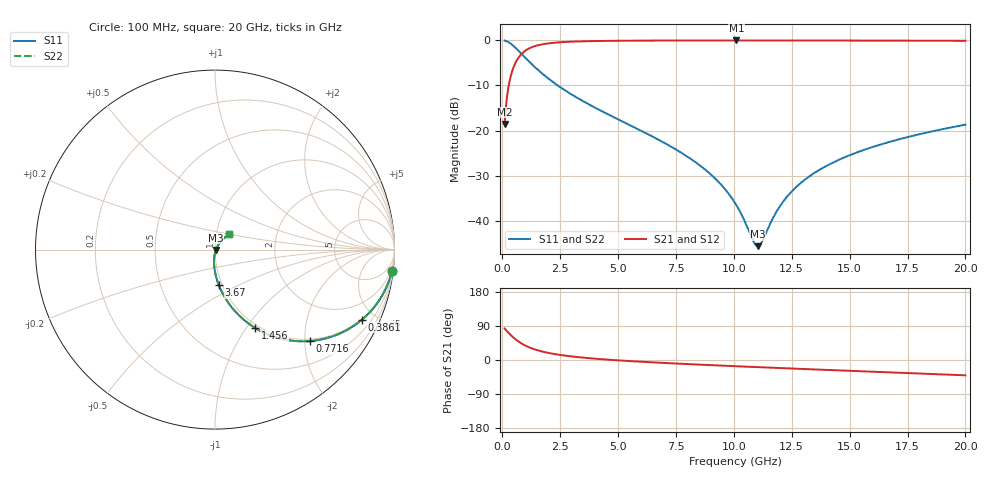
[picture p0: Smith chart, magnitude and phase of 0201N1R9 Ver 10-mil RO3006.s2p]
# GHz S MA R 50
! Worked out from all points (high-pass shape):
!   1601 points, 100 MHz to 20 GHz, reference 50 ohm
!   highest |S21| = -0.05 dB at 10.11 GHz (marker M1); lowest = -18.5 dB at 100 MHz (marker M2)
!   |S21| within 3 dB of the highest: 828.2 MHz to end of sweep
!   lowest |S11| = -45.5 dB at 11.03 GHz (marker M3), VSWR 1.01, Z = 50.5 - j0.181 ohm
!   |S11| at or under -10 dB: 2.395 GHz to end of sweep
!   |S22| runs from -45.5 to -0.1 dB; largest |S21 - S12| = 0
!   S11 on the Smith chart (normalised r, x): 100 MHz: 1, -16; 386.1 MHz: 0.96, -4.23; 771.6 MHz: 0.96, -2.11; 1.456 GHz: 0.96, -1.10; 3.67 GHz: 0.96, -0.40; 20 GHz: 1.16, +0.20
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0.1  0.9929 -7.0  0.1186 83.0  0.1186 83.0  0.9929 -7.0
0.2616875  0.9542 -17.8  0.2983 72.1  0.2983 72.1  0.9542 -17.8
0.3860625  0.9076 -25.4  0.4189 64.5  0.4189 64.5  0.9076 -25.4
0.771625  0.733 -44.1  0.6785 45.8  0.6785 45.8  0.733 -44.1
1.095  0.6029 -54.6  0.7956 35.2  0.7956 35.2  0.6029 -54.6
1.455688  0.4915 -62.8  0.8683 26.9  0.8683 26.9  0.4915 -62.8
2.226812  0.3393 -73.5  0.9376 16.0  0.9376 16.0  0.3393 -73.5
3.420812  0.2168 -82.4  0.9727 6.6  0.9727 6.6  0.2168 -82.4
3.669563  0.1998 -83.8  0.9762 5.2  0.9762 5.2  0.1998 -83.8
6.741625  0.07955 -93.9  0.9923 -7.0  0.9923 -7.0  0.07955 -93.9
8.781375  0.03676 -95.4  0.9943 -13.0  0.9943 -13.0  0.03676 -95.4
10.05  0.01588 -87.6  0.9945 -16.3  0.9945 -16.3  0.01588 -87.6
10.11219  0.01496 -86.5  0.9945 -16.5  0.9945 -16.5  0.01496 -86.5
10.846  0.005969 -46.8  0.9945 -18.4  0.9945 -18.4  0.005969 -46.8
11.03256  0.005285 -19.8  0.9944 -18.9  0.9944 -18.9  0.005285 -19.8
11.20669  0.005856 5.5  0.9944 -19.3  0.9944 -19.3  0.005856 5.5
11.72906  0.0113 40.8  0.9942 -20.6  0.9942 -20.6  0.0113 40.8
12.16437  0.01689 49.3  0.9941 -21.7  0.9941 -21.7  0.01689 49.3
13.37081  0.03268 55.3  0.9934 -24.6  0.9934 -24.6  0.03268 55.3
14.78869  0.05083 55.2  0.9924 -28.0  0.9924 -28.0  0.05083 55.2
16.69162  0.07474 52.6  0.9905 -32.6  0.9905 -32.6  0.07474 52.6
20  0.1166 46.2  0.9858 -40.4  0.9858 -40.4  0.1166 46.2
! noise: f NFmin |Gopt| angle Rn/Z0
0.1  0.0009637  0.9565  0.6645  0.00499
2.301  0.005358  0.826  4.33  0.006463
4.515  0.008286  0.7844  8.032  0.007855
6.729  0.01081  0.7577  11.73  0.008937
8.943  0.01311  0.7383  15.41  0.009853
11.14  0.01527  0.7233  19.05  0.01066
13.36  0.01735  0.7113  22.66  0.0114
15.57  0.01937  0.7016  26.24  0.01208
17.79  0.02134  0.6938  29.77  0.01273
20  0.0233  0.6875  33.25  0.01334
